| TEXAS INSTRUMENTS INCORPORATED
| Standard Linear and Logic Group
| IBIS Model of PCA9539
| REMOTE 16-BIT I2C AND SMBus LOW-POWER I/O EXPANDER WITH INTERRUPT
| OUTPUT, RESET, AND CONFIGURATION REGISTERS
| This file contains package information for the following:
|  SSOP 24-pin (DB) package as [Component] PCA9539_DB
|  SSOP 24-pin (DBQ) package as [Component] PCA9539_DBQ
|  TVSOP 24-pin (DGV) package as [Component] PCA9539_DGV
|  SOIC 24-pin (DW) package as [Component] PCA9539_DW
|  TSSOP 24-pin (PW) package as [Component] PCA9539_PW
|  QFN 24-pin (RGE) package as [Component] PCA9539_RGE
| This device can be powered at the following Vccs:
|  5 volt Vcc
|  3.3 volt Vcc
|  2.5 volt Vcc
| This file provides unique models under the [Model Selector] for each Vcc.
| For operation at a specific Vcc, select the appropriate model after each
| [Model Selector] keyword.
[IBIS Ver]   3.2
[Comment char]  |_char
[File Name]   pca9539.ibs
[File Rev]   1.1 | x_die
[Date]   May 3, 2007
[Source]   Data created from TI-SPICE simulations at TI-SLL.
[Notes]   The following is an IBIS list for the PCA9539.
   Please contact sllibis@ti.com with questions and
   comments concerning SLL IBIS models.
   - FILE REV HISTORY
   - 1.1 Release IBIS file on 05/09/07
   - Power clamp data has been deleted in the SCL, P, SDA,
   and INT, models as there is no power-clamp diode.
   - End point warning due to AC and DC mismatch.
[Disclaimer] Property of Texas Instruments Incorporated.  Unauthorized
   reproduction and/or distribution is strictly prohibited.
   This product is protected under copyright law.
   Created  2007, (C) Copyright  2007, Texas Instruments
   Incorporated, All Rights Reserved
   UNLESS THERE IS A SIGNED, WRITTEN AGREEMENT TO THE
   CONTRARY, TEXAS INSTRUMENTS (TI) IS PROVIDING THE IBIS
   MODELS  AND WITHOUT ANY WARRANTY, EXPRESSED OR
   IMPLIED.  TI assumes no liability for:
   1) the accuracy of the IBIS models provided to your
   company;
   2) the proper functioning of these IBIS Models in your
   design or for any resulting applications; or
   3) infringement of patents, copyrights or intellectual
   property rights resulting from your use of these IBIS
   models.
   TI provides IBIS Models as a service to our customers.
   You and your company shall not distribute, sell or give
   these models to anyone else without prior written
   permission from TI.
   TI reserves the right to make changes to our products or
   to discontinue any semiconductor product or service
   without notice, and advises our customers to obtain the
   latest version of relevant information to verify, before
   placing orders, that the information being relied on is
   current.
   Please be aware that your receipt and use of the IBIS
   information provided shall serve as acceptance of these
   terms and conditions.  If you do not accept these terms,
   you should return or destroy the IBIS models and any
   other accompanying information immediately.
| Component PCA9539_DB 24-PIN SSOP
[Component]   PCA9539_DB
[Manufacturer]   Texas Instruments, Inc.
[Package]
|   typ   min   max
R_pkg   4.500e-02   4.000e-02   4.900e-02
L_pkg   3.668e-09   3.226e-09   4.415e-09
C_pkg   4.160e-13   3.490e-13   5.070e-13
[Pin]   signal_name   model_name   R_pin   L_pin   C_pin
1   NINT   PCA9539_INT   4.200e-02   4.299e-09   5.030e-13
2   A1   PCA9539_A   4.000e-02   3.960e-09   4.990e-13
3   NRESET   NC   4.200e-02   3.775e-09   4.170e-13
4   P00   PCA9539_P   4.700e-02   3.487e-09   3.690e-13
5   P01   PCA9539_P   4.600e-02   3.347e-09   3.520e-13
6   P02   PCA9539_P   4.900e-02   3.352e-09   3.710e-13
7   P03   PCA9539_P   4.600e-02   3.226e-09   3.630e-13
8   P04   PCA9539_P   4.700e-02   3.289e-09   3.490e-13
9   P05   PCA9539_P   4.700e-02   3.347e-09   3.610e-13
10   P06   PCA9539_P   4.100e-02   3.576e-09   4.090e-13
11   P07   PCA9539_P   4.100e-02   3.995e-09   5.030e-13
12   GND   GND   4.500e-02   4.415e-09   5.070e-13
13   P10   PCA9539_P   4.300e-02   4.337e-09   5.060e-13
14   P11   PCA9539_P   4.200e-02   4.003e-09   5.040e-13
15   P12   PCA9539_P   4.100e-02   3.686e-09   4.100e-13
16   P13   PCA9539_P   4.800e-02   3.355e-09   3.490e-13
17   P14   PCA9539_P   4.700e-02   3.301e-09   3.530e-13
18   P15   PCA9539_P   4.800e-02   3.268e-09   3.660e-13
19   P16   PCA9539_P   4.800e-02   3.269e-09   3.660e-13
20   P17   PCA9539_P   4.700e-02   3.314e-09   3.490e-13
21   A0   PCA9539_A   4.800e-02   3.399e-09   3.550e-13
22   SCL   PCA9539_SCL   4.100e-02   3.688e-09   4.120e-13
23   SDA   PCA9539_SDA   4.200e-02   4.003e-09   5.040e-13
24   VCC   POWER   4.300e-02   4.347e-09   5.050e-13
| Component PCA9539_DBQ 24-PIN SSOP
[Component]   PCA9539_DBQ
[Manufacturer]   Texas Instruments, Inc.
[Package]
|   typ   min   max
R_pkg   4.400e-02   3.100e-02   6.600e-02
L_pkg   3.074e-09   2.348e-09   4.044e-09
C_pkg   3.220e-13   2.340e-13   4.460e-13
[Pin]   signal_name   model_name   R_pin   L_pin   C_pin
1   NINT   PCA9539_INT   6.500e-02   4.044e-09   4.290e-13
2   A1   PCA9539_A   6.600e-02   3.824e-09   4.460e-13
3   NRESET   NC   3.100e-02   3.011e-09   3.210e-13
4   P00   PCA9539_P   3.200e-02   2.699e-09   2.590e-13
5   P01   PCA9539_P   3.500e-02   2.519e-09   2.450e-13
6   P02   PCA9539_P   3.500e-02   2.348e-09   2.340e-13
7   P03   PCA9539_P   3.500e-02   2.348e-09   2.340e-13
8   P04   PCA9539_P   3.500e-02   2.518e-09   2.450e-13
9   P05   PCA9539_P   3.200e-02   2.699e-09   2.590e-13
10   P06   PCA9539_P   3.100e-02   3.011e-09   3.210e-13
11   P07   PCA9539_P   6.600e-02   3.824e-09   4.460e-13
12   GND   GND   6.500e-02   4.044e-09   4.290e-13
13   P10   PCA9539_P   6.500e-02   4.044e-09   4.290e-13
14   P11   PCA9539_P   6.600e-02   3.824e-09   4.460e-13
15   P12   PCA9539_P   3.100e-02   3.011e-09   3.210e-13
16   P13   PCA9539_P   3.200e-02   2.699e-09   2.590e-13
17   P14   PCA9539_P   3.500e-02   2.518e-09   2.450e-13
18   P15   PCA9539_P   3.500e-02   2.348e-09   2.340e-13
19   P16   PCA9539_P   3.500e-02   2.348e-09   2.340e-13
20   P17   PCA9539_P   3.500e-02   2.518e-09   2.450e-13
21   A0   PCA9539_A   3.200e-02   2.699e-09   2.590e-13
22   SCL   PCA9539_SCL   3.100e-02   3.011e-09   3.210e-13
23   SDA   PCA9539_SDA   6.600e-02   3.824e-09   4.460e-13
24   VCC   POWER   6.500e-02   4.044e-09   4.290e-13
| Component PCA9539_DGV 24-PIN TVSOP
[Component]   PCA9539_DGV
[Manufacturer]   Texas Instruments, Inc.
[Package]
|   typ   min   max
R_pkg   4.300e-02   3.900e-02   4.700e-02
L_pkg   2.601e-09   2.312e-09   3.626e-09
C_pkg   3.580e-13   2.770e-13   5.950e-13
[Pin]   signal_name   model_name   R_pin   L_pin   C_pin
1   NINT   PCA9539_INT   4.300e-02   3.625e-09   5.950e-13
2   A1   PCA9539_A   4.000e-02   2.656e-09   4.020e-13
3   NRESET   NC   3.900e-02   2.338e-09   3.080e-13
4   P00   PCA9539_P   4.600e-02   2.354e-09   2.770e-13
5   P01   PCA9539_P   4.500e-02   2.312e-09   2.850e-13
6   P02   PCA9539_P   4.700e-02   2.318e-09   2.820e-13
7   P03   PCA9539_P   4.700e-02   2.318e-09   2.820e-13
8   P04   PCA9539_P   4.500e-02   2.312e-09   2.850e-13
9   P05   PCA9539_P   4.600e-02   2.353e-09   2.780e-13
10   P06   PCA9539_P   3.900e-02   2.338e-09   3.080e-13
11   P07   PCA9539_P   4.100e-02   2.660e-09   4.020e-13
12   GND   GND   4.300e-02   3.625e-09   5.950e-13
13   P10   PCA9539_P   4.400e-02   3.626e-09   5.940e-13
14   P11   PCA9539_P   4.000e-02   2.658e-09   4.020e-13
15   P12   PCA9539_P   3.900e-02   2.343e-09   3.110e-13
16   P13   PCA9539_P   4.600e-02   2.353e-09   2.780e-13
17   P14   PCA9539_P   4.500e-02   2.312e-09   2.850e-13
18   P15   PCA9539_P   4.700e-02   2.319e-09   2.820e-13
19   P16   PCA9539_P   4.700e-02   2.319e-09   2.820e-13
20   P17   PCA9539_P   4.500e-02   2.312e-09   2.850e-13
21   A0   PCA9539_A   4.600e-02   2.353e-09   2.780e-13
22   SCL   PCA9539_SCL   3.900e-02   2.337e-09   3.080e-13
23   SDA   PCA9539_SDA   4.000e-02   2.658e-09   4.020e-13
24   VCC   POWER   4.400e-02   3.626e-09   5.950e-13
| Component PCA9539_DW 24-PIN SOIC
[Component]   PCA9539_DW
[Manufacturer]   Texas Instruments, Inc.
[Package]
|   typ   min   max
R_pkg   3.700e-02   3.000e-02   4.700e-02
L_pkg   5.146e-09   3.993e-09   6.885e-09
C_pkg   7.580e-13   5.120e-13   1.067e-12
[Pin]   signal_name   model_name   R_pin   L_pin   C_pin
1   NINT   PCA9539_INT   3.900e-02   6.885e-09   1.067e-12
2   A1   PCA9539_A   4.200e-02   5.950e-09   9.580e-13
3   NRESET   NC   4.700e-02   5.317e-09   7.910e-13
4   P00   PCA9539_P   3.100e-02   4.651e-09   6.110e-13
5   P01   PCA9539_P   3.000e-02   3.993e-09   5.120e-13
6   P02   PCA9539_P   3.000e-02   4.083e-09   6.110e-13
7   P03   PCA9539_P   3.000e-02   4.083e-09   6.110e-13
8   P04   PCA9539_P   3.000e-02   3.993e-09   5.120e-13
9   P05   PCA9539_P   3.100e-02   4.652e-09   6.110e-13
10   P06   PCA9539_P   4.700e-02   5.317e-09   7.910e-13
11   P07   PCA9539_P   4.200e-02   5.950e-09   9.590e-13
12   GND   GND   3.900e-02   6.885e-09   1.067e-12
13   P10   PCA9539_P   3.900e-02   6.885e-09   1.067e-12
14   P11   PCA9539_P   4.200e-02   5.950e-09   9.590e-13
15   P12   PCA9539_P   4.700e-02   5.317e-09   7.910e-13
16   P13   PCA9539_P   3.100e-02   4.652e-09   6.110e-13
17   P14   PCA9539_P   3.000e-02   3.993e-09   5.120e-13
18   P15   PCA9539_P   3.000e-02   4.083e-09   6.100e-13
19   P16   PCA9539_P   3.000e-02   4.083e-09   6.100e-13
20   P17   PCA9539_P   3.000e-02   3.993e-09   5.120e-13
21   A0   PCA9539_A   3.100e-02   4.651e-09   6.110e-13
22   SCL   PCA9539_SCL   4.700e-02   5.317e-09   7.910e-13
23   SDA   PCA9539_SDA   4.200e-02   5.950e-09   9.580e-13
24   VCC   POWER   3.900e-02   6.885e-09   1.067e-12
| Component PCA9539_PW 24-PIN TSSOP
[Component]   PCA9539_PW
[Manufacturer]   Texas Instruments, Inc.
[Package]
|   typ   min   max
R_pkg   3.900e-02   3.000e-02   4.600e-02
L_pkg   2.685e-09   2.367e-09   3.177e-09
C_pkg   3.200e-13   2.520e-13   4.340e-13
[Pin]   signal_name   model_name   R_pin   L_pin   C_pin
1   NINT   PCA9539_INT   3.700e-02   3.153e-09   4.340e-13
2   A1   PCA9539_A   3.400e-02   2.629e-09   3.410e-13
3   NRESET   NC   3.200e-02   2.860e-09   3.470e-13
4   P00   PCA9539_P   4.200e-02   2.741e-09   2.900e-13
5   P01   PCA9539_P   4.600e-02   2.600e-09   2.620e-13
6   P02   PCA9539_P   4.300e-02   2.414e-09   2.660e-13
7   P03   PCA9539_P   4.200e-02   2.367e-09   2.620e-13
8   P04   PCA9539_P   4.400e-02   2.461e-09   2.520e-13
9   P05   PCA9539_P   4.200e-02   2.543e-09   2.740e-13
10   P06   PCA9539_P   3.000e-02   2.616e-09   3.320e-13
11   P07   PCA9539_P   3.700e-02   2.670e-09   3.460e-13
12   GND   GND   3.900e-02   3.177e-09   4.330e-13
13   P10   PCA9539_P   3.700e-02   3.111e-09   4.310e-13
14   P11   PCA9539_P   3.700e-02   2.656e-09   3.450e-13
15   P12   PCA9539_P   3.100e-02   2.739e-09   3.400e-13
16   P13   PCA9539_P   4.200e-02   2.649e-09   2.820e-13
17   P14   PCA9539_P   4.600e-02   2.532e-09   2.570e-13
18   P15   PCA9539_P   4.400e-02   2.425e-09   2.660e-13
19   P16   PCA9539_P   4.400e-02   2.425e-09   2.660e-13
20   P17   PCA9539_P   4.600e-02   2.532e-09   2.570e-13
21   A0   PCA9539_A   4.200e-02   2.648e-09   2.820e-13
22   SCL   PCA9539_SCL   3.100e-02   2.738e-09   3.390e-13
23   SDA   PCA9539_SDA   3.600e-02   2.653e-09   3.440e-13
24   VCC   POWER   3.700e-02   3.110e-09   4.310e-13
| Component PCA9539_RGE 24-PIN QFN
[Component]   PCA9539_RGE
[Manufacturer]   Texas Instruments, Inc.
[Package]
|   typ   min   max
R_pkg   3.700e-02   2.500e-02   5.300e-02
L_pkg   8.060e-10   5.310e-10   1.139e-09
C_pkg   1.880e-13   5.700e-14   3.100e-13
[Pin]   signal_name   model_name   R_pin   L_pin   C_pin
1   P00   PCA9539_P   3.300e-02   7.260e-10   2.460e-13
2   P01   PCA9539_P   3.200e-02   6.830e-10   2.620e-13
3   P02   PCA9539_P   3.000e-02   6.550e-10   2.410e-13
4   P03   PCA9539_P   3.000e-02   6.580e-10   2.400e-13
5   P04   PCA9539_P   3.100e-02   6.770e-10   2.330e-13
6   P05   PCA9539_P   3.500e-02   7.590e-10   2.490e-13
7   P06   PCA9539_P   3.700e-02   7.990e-10   2.540e-13
8   P07   PCA9539_P   4.500e-02   9.840e-10   2.710e-13
9   GND   GND   4.500e-02   9.870e-10   2.580e-13
10   P10   PCA9539_P   4.100e-02   8.860e-10   2.340e-13
11   P11   PCA9539_P   4.700e-02   1.014e-09   2.510e-13
12   P12   PCA9539_P   3.600e-02   7.740e-10   2.390e-13
13   P13   PCA9539_P   3.600e-02   7.870e-10   2.540e-13
14   P14   PCA9539_P   3.200e-02   7.070e-10   2.350e-13
15   P15   PCA9539_P   2.900e-02   6.430e-10   2.300e-13
16   P16   PCA9539_P   3.000e-02   6.450e-10   2.300e-13
17   P17   PCA9539_P   3.300e-02   7.100e-10   2.360e-13
18   A0   PCA9539_A   3.800e-02   8.150e-10   2.570e-13
19   SCL   PCA9539_SCL   3.600e-02   7.750e-10   2.390e-13
20   SDA   PCA9539_SDA   4.700e-02   1.015e-09   2.510e-13
21   VCC   POWER   4.100e-02   8.850e-10   2.360e-13
22   NINT   PCA9539_INT   4.700e-02   1.028e-09   3.100e-13
23   A1   PCA9539_A   5.300e-02   1.139e-09   2.800e-13
24   NRESET   NC   3.400e-02   7.350e-10   2.480e-13
| Model PCA9539_A
[Model Selector]   PCA9539_A
PCA9539_A_50   5 volt Vcc
PCA9539_A_33   3.3 volt Vcc
PCA9539_A_25   2.5 volt Vcc
| Model PCA9539_SCL
[Model Selector]   PCA9539_SCL
PCA9539_SCL_50   5 volt Vcc
PCA9539_SCL_33   3.3 volt Vcc
PCA9539_SCL_25   2.5 volt Vcc
| Model PCA9539_P
[Model Selector]   PCA9539_P
PCA9539_P_50   5 volt Vcc
PCA9539_P_33   3.3 volt Vcc
PCA9539_P_25   2.5 volt Vcc
| Model PCA9539_SDA
[Model Selector]   PCA9539_SDA
PCA9539_SDA_50   5 volt Vcc
PCA9539_SDA_33   3.3 volt Vcc
PCA9539_SDA_25   2.5 volt Vcc
| Model PCA9539_INT
[Model Selector]   PCA9539_INT
PCA9539_INT_50   5 volt Vcc
PCA9539_INT_33   3.3 volt Vcc
PCA9539_INT_25   2.5 volt Vcc
| Models and submodels in the file (15): PCA9539_A_50 (Input), PCA9539_A_33 (Input), PCA9539_A_25 (Input), PCA9539_SCL_50 (Input), PCA9539_SCL_33 (Input), PCA9539_SCL_25 (Input), PCA9539_P_50 (I/O), PCA9539_P_33 (I/O), PCA9539_P_25 (I/O), PCA9539_SDA_50 (I/O_open_drain), PCA9539_SDA_33 (I/O_open_drain), PCA9539_SDA_25 (I/O_open_drain), PCA9539_INT_50 (Open_drain), PCA9539_INT_33 (Open_drain), PCA9539_INT_25 (Open_drain)
